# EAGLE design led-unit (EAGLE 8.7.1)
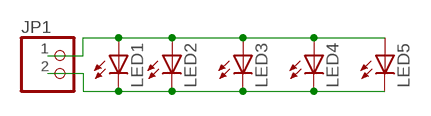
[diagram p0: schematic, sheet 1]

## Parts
JP1  PINHD-1X02_2.54-SMD  [1X02SMD]
LED1  LED3MM  [LED3MM]
LED2  LED3MM  [LED3MM]
LED3  LED3MM  [LED3MM]
LED4  LED3MM  [LED3MM]
LED5  LED3MM  [LED3MM]

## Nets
N$1: JP1.1 LED1.A LED2.A LED3.A LED4.A LED5.A
N$2: JP1.2 LED1.K(C) LED2.K(C) LED3.K(C) LED4.K(C) LED5.K(C)

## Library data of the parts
JP1 = pinhead-2:PINHD-1X02: PIN HEADER
LED1-LED5 = led:LED: LED

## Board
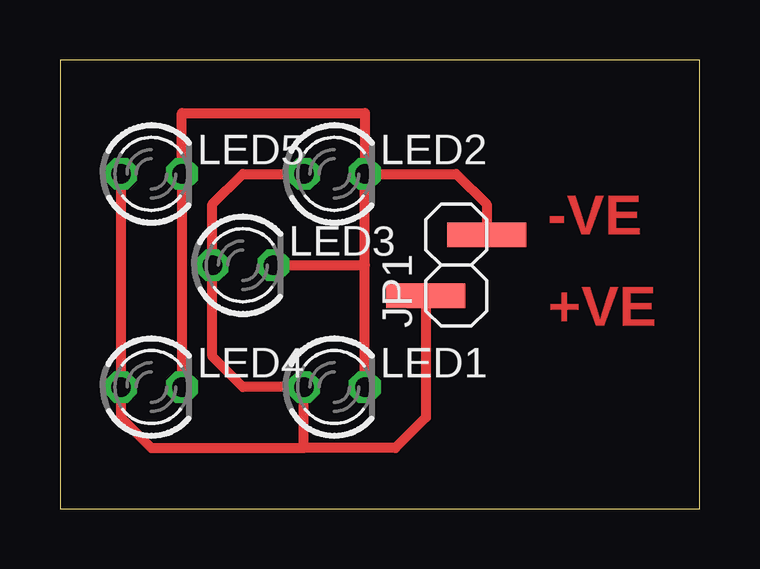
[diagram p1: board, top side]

Size 26.65 x 18.72 mm. Coordinates in mm from the lower left corner, seen from the top.
Outline: 0,0 26.65,0 26.65,18.72 0,18.72 0,0
Copper layers (1*16): Top 0.035mm / dielectric 1.5mm / Bottom 0.035mm
Design rules "default *": minimum track width 16mil, minimum drill 0.35mm, track to track 16mil, track to pad 16mil, pad to pad 16mil, via to via 16mil, smd to smd 16mil, copper to edge 40mil, drill to drill 6mil, minimum pad ring 10mil, minimum via ring 8mil, stop-mask expansion 4mil, vias tented up to drill 0mil, thermal gap 10mil

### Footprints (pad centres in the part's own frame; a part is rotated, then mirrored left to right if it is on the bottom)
1X02SMD = smd 1.016 x 3.302: 1 -1.27,1.27; 2 1.27,-1.27
LED3MM = drill 0.813 octagon: A -1.27,0; K 1.27,0

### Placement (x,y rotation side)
JP1  16.51,10.16 90 top
LED1  11.43,5.08 0 top
LED2  11.43,13.97 0 top
LED3  7.62,10.16 0 top
LED4  3.81,5.08 0 top
LED5  3.81,13.97 0 top

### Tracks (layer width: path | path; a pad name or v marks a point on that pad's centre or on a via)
N$1
  Top 0.406: LED5.A LED4.A 2.54,3.81 3.81,2.54 10.16,2.54 | 10.16,2.54 13.97,2.54 15.24,3.81 JP1.1 | 10.16,2.54 LED1.A 7.62,5.08 6.35,6.35 LED3.A 6.35,12.7 7.62,13.97 LED2.A
N$2
  Top 0.406: LED4.K LED5.K 5.08,16.51 12.7,16.51 LED2.K | LED2.K 16.51,13.97 17.78,12.7 JP1.2 | LED1.K 12.7,10.16 | 12.7,10.16 LED2.K | LED3.K 12.7,10.16

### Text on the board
Top: -VE | +VE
